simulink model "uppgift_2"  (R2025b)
settings: Solver=VariableStepAuto  StartTime=0.0  StopTime=10.0  RelTol=1e-3
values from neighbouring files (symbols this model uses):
  m_th_1 = 12/1000    (= 0.012)    [Lektion_2.m]
  m_th_2 = 16/1000    (= 0.016)    [Lektion_2.m]
  tau_th = 1/0.1    (= 10)    [Lektion_2.m]

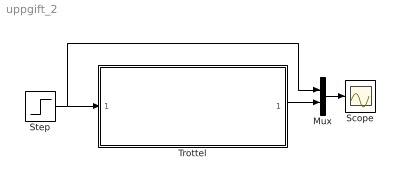
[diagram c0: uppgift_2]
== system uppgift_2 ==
  Mux : Mux  Inputs=2
  Scope : Scope
  Step : Step  Time=2  Before=m_th_1  After=m_th_2  SampleTime=0
  Trottel : Subsystem
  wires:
  Step/1 -> Mux/1, Trottel/1(m_at,raf [kg/s])
  Mux/1 -> Scope/1
  Trottel/1(m_at [kg/s]) -> Mux/2

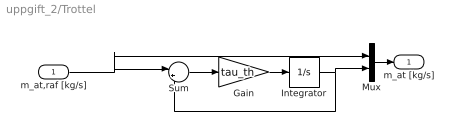
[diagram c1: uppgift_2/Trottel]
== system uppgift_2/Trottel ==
  m_at,raf [kg/s] : Inport
  Gain : Gain  Gain=tau_th
  Integrator : Integrator  InitialCondition=m_th_1
  Mux : Mux  Inputs=2
  Sum : Sum  Inputs=|+-
  m_at [kg/s] : Outport
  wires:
  Sum/1 -> Gain/1
  Integrator/1 -> Sum/2, Mux/2
  Mux/1 -> m_at [kg/s]/1
  m_at,raf [kg/s]/1 -> Sum/1, Mux/1
  Gain/1 -> Integrator/1
